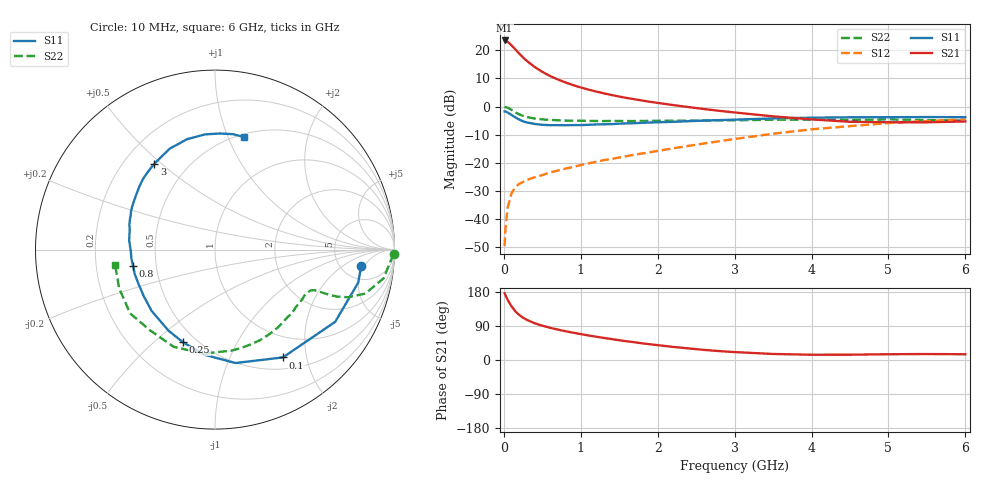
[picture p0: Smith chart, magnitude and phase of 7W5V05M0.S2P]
! Infineon Technologies  Discrete & RF Semiconductors
! BFS17W
! Si NPN RF Bipolar Junction Transistor in SOT323
! VCE = 5 V  IC = 5 mA
! Common Emitter S-Parameters:  August  1999
# GHz  S  MA  R  50
!  f  S11  S21  S12  S22
! GHz  MAG  ANG  MAG  ANG  MAG  ANG  MAG  ANG
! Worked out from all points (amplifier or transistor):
!   36 points, 10 MHz to 6 GHz, reference 50 ohm
!   highest |S21| = 23.5 dB at 10 MHz (marker M1)
!   |S21| within 3 dB of that: start of sweep to 143.4 MHz
!   unconditionally stable (mu >= 1): 570.7 MHz to 2.544 GHz; 4.722 GHz to end of sweep
!   at 250 MHz: K = 0.58, MSG = 22.1 dB, |S12| = -26.8 dB
!   at 1.4 GHz: K = 1.23, MAG = 8.5 dB, |S12| = -18.6 dB
!   at 6 GHz: K = 1.07, MAG = -2.0 dB, |S12| = -4.5 dB
!   S11 on the Smith chart (normalised r, x): 10 MHz: 7.71, -4.21; 100 MHz: 0.66, -1.61; 250 MHz: 0.42, -0.62; 800 MHz: 0.37, -0.08; 3 GHz: 0.33, +0.47; 6 GHz: 0.53, +1.14
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0.01  0.8188 -6.3  14.96 176.1  0.0033 79.9  0.9957 -1.5
0.02  0.8191 -12.9  14.82 171.3  0.0066 89.3  0.9785 -4.0
0.05  0.7813 -31.0  14.16 158.7  0.016 74.1  0.9538 -9.6
0.1  0.7099 -57.8  12.29 141.7  0.0288 64.1  0.8727 -16.3
0.15  0.6421 -79.8  10.35 128.3  0.0369 55.1  0.7874 -19.7
0.2  0.5883 -96.0  8.743 118.9  0.0424 53.0  0.7265 -21.1
0.25  0.546 -109.1  7.443 111.6  0.0457 49.9  0.681 -21.6
0.3  0.5208 -119.8  6.458 105.9  0.0495 49.3  0.6521 -21.8
0.4  0.4913 -136.0  5.062 97.0  0.0554 49.6  0.6124 -22.0
0.5  0.4739 -147.2  4.145 90.5  0.0607 51.5  0.5923 -22.4
0.6  0.467 -155.9  3.496 85.0  0.0671 53.3  0.579 -23.2
0.8  0.4653 -168.9  2.689 76.0  0.0788 56.7  0.565 -25.9
0.9  0.4685 -173.9  2.405 72.1  0.0844 58.2  0.5596 -27.5
1.1  0.4742 177.4  2.002 64.7  0.098 60.7  0.5567 -31.4
1.3  0.4842 169.8  1.72 58.2  0.1117 62.8  0.5528 -35.8
1.6  0.5027 160.6  1.419 49.4  0.1318 64.7  0.5525 -42.7
2.2  0.5356 144.9  1.064 34.6  0.1809 68.0  0.5607 -58.3
3  0.5855 125.3  0.785 20.9  0.2649 67.1  0.5703 -80.8
3.5  0.6161 114.3  0.67 15.9  0.3289 63.8  0.5824 -96.1
4.5  0.6442 95.0  0.536 14.0  0.4489 51.9  0.5772 -128.6
5.5  0.651 81.1  0.525 15.7  0.5536 39.0  0.5758 -158.1
6  0.6474 75.7  0.544 15.2  0.5946 32.6  0.563 -171.2
